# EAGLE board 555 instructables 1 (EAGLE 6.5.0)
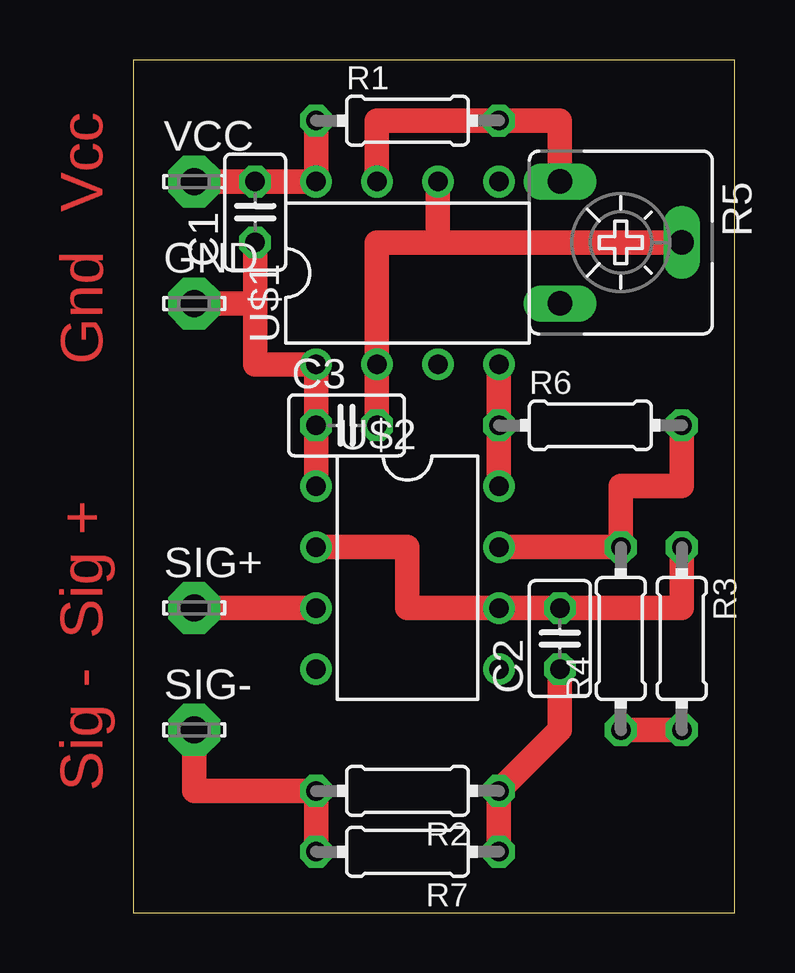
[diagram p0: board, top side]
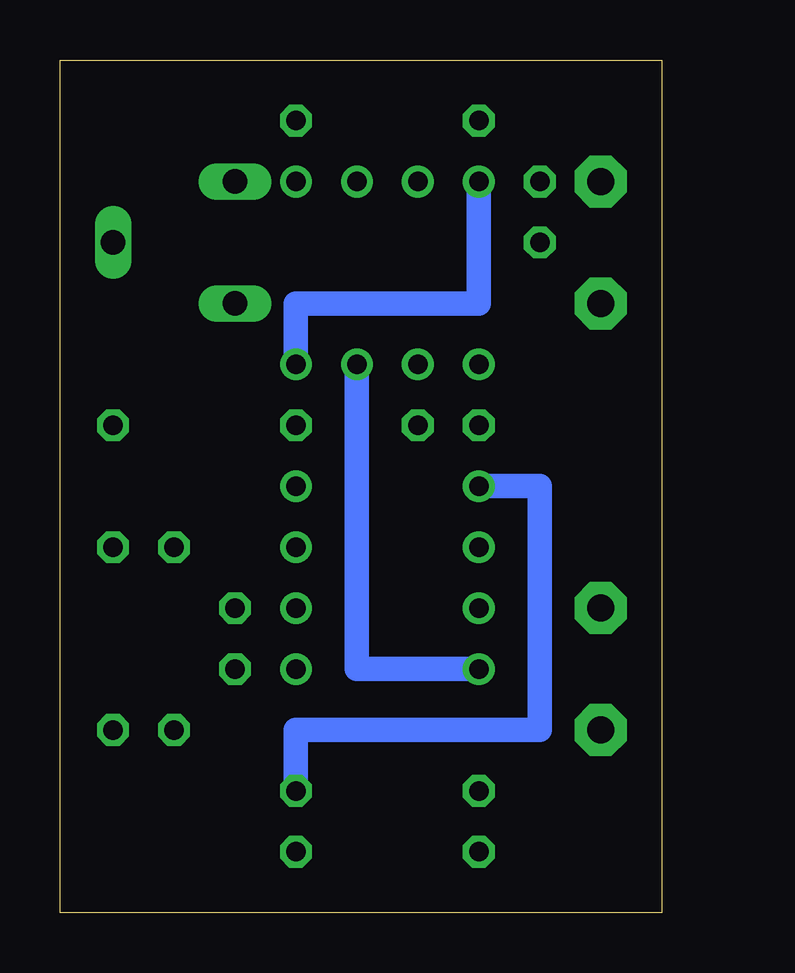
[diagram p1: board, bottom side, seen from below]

Size 25.07 x 35.55 mm. Coordinates in mm from the lower left corner, seen from the top.
Outline: 0,0 25.07,0 25.07,35.55 0,35.55 0,0
Copper layers (1*16): Top 0.035mm / dielectric 1.5mm / Bottom 0.035mm
Design rules "default": minimum track width 10mil, minimum drill 24mil, track to track 8mil, track to pad 8mil, pad to pad 8mil, via to via 8mil, smd to smd 8mil, copper to edge 40mil, drill to drill 8mil, minimum pad ring 10mil, minimum via ring 8mil, stop-mask expansion 4mil, vias tented up to drill 0mil, thermal gap 10mil

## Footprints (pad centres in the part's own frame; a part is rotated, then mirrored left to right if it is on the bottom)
C025-025X050 = drill 0.813 octagon: 1 -1.27,0; 2 1.27,0
LSP11 = drill 1.118 pad 2.159 octagon: MP 0,0
0204/7 = drill 0.813 octagon: 1 -3.81,0; 2 3.81,0
CA6V = drill 1.016 long: A -2.54,-2.54; E 2.54,-2.54; S 0,2.54
DIL8 = drill 0.813 pad 1.27: 1 -5.08,-2.54; 2 -2.54,-2.54; 3 0,-2.54; 4 2.54,-2.54; 5 2.54,5.08; 6 0,5.08; 7 -2.54,5.08; 8 -5.08,5.08

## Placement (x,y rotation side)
C1  10uF  [C025-025X050]  5.08,29.21 90 top
C2  .01uF  [C025-025X050]  17.78,11.43 90 top
C3  .1uF  [C025-025X050]  8.89,20.32 0 top
GND  LSP11  [LSP11]  2.54,25.4 0 top
R1  1K  [0204/7]  11.43,33.02 0 top
R2  100  [0204/7]  11.43,5.08 180 top
R3  1K  [0204/7]  22.86,11.43 270 top
R4  5.6K  [0204/7]  20.32,11.43 90 top
R5  500K  [CA6V]  20.32,27.94 270 top
R6  1K  [0204/7]  19.05,20.32 0 top
R7  100  [0204/7]  11.43,2.54 180 top
SIG+  LSP11  [LSP11]  2.54,12.7 0 top
SIG-  LSP11  [LSP11]  2.54,7.62 0 top
U$1  LM555  [DIL8]  12.7,25.4 0 top
U$2  LM555  [DIL8]  10.16,12.7 270 top
VCC  LSP11  [LSP11]  2.54,30.48 0 top

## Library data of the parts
C1-C3 R1-R4 R6 R7 = rcl
GND SIG+ SIG- VCC = solpad
R5 = pot
U$1 U$2 = john

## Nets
N$1: C3.2 R5.S U$1.2 U$1.6
N$2: SIG+.MP U$2.3
N$3: U$1.3 U$2.4
N$4: C2.2 R3.1 U$2.2 U$2.6
N$5: C1.2 R1.1 R6.1 U$1.4 U$1.8 U$2.8 VCC.MP
N$6: R1.2 R5.A U$1.7
N$7: R2.2 R7.2 SIG-.MP
N$8: R3.2 R4.1
N$9: R4.2 R6.2 U$2.7
N$13: C1.1 C2.1 C3.1 GND.MP R2.1 R7.1 U$1.1 U$2.1

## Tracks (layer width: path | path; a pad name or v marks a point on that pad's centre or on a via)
N$1
  Top 1.016: R5.S 12.7,27.94 | 12.7,27.94 U$1.6 | 12.7,27.94 10.16,27.94 U$1.2 C3.2
N$2
  Top 1.016: U$2.3 SIG+.MP
N$3
  Bottom 1.016: U$1.3 12.7,10.16 U$2.4
N$4
  Top 1.016: U$2.2 11.43,15.24 11.43,12.7 U$2.6 C2.2 22.86,12.7 R3.1
N$5
  Top 1.016: U$2.8 R6.1 U$1.4 | VCC.MP C1.2 U$1.8 R1.1
  Bottom 1.016: U$1.8 7.62,25.4 15.24,25.4 U$1.4
N$6
  Top 1.016: R5.A 17.78,33.02 R1.2 10.16,33.02 U$1.7
N$7
  Top 1.016: R7.2 R2.2 2.54,5.08 SIG-.MP
N$8
  Top 1.016: R3.2 R4.1
N$9
  Top 1.016: U$2.7 R4.2 20.32,17.78 22.86,17.78 R6.2
N$13
  Top 1.016: GND.MP 5.08,25.4 | 5.08,25.4 5.08,22.86 U$1.1 C3.1 U$2.1 | C1.1 5.08,25.4 | C2.1 17.78,7.62 R2.1 R7.1
  Bottom 1.016: U$2.1 5.08,17.78 5.08,7.62 15.24,7.62 R2.1

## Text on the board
Top: Vcc | Gnd | Sig + | Sig -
